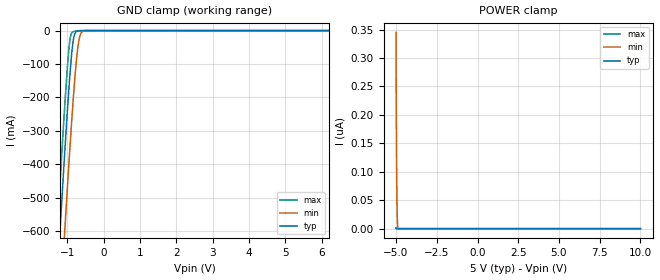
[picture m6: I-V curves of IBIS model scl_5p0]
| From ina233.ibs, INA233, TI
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|   scl_5p0
[Model]   scl_5p0
Model_type   Input
Vinl = 0.4
Vinh = 3.5
|   typ   min   max
C_comp   6.141E-13   5.923E-13   6.345E-13
| Where Nom  PVT is Nominal Process, 5V, 25C
|   Fast PVT is Strong Process,  5.5V, -40C
|   Slow PVT is Weak Process,   4.5V, 125C
[Voltage Range]   5   4.5   5.5
[Temperature Range]   25   125   -40
[Power Clamp Reference]   5   4.5   5.5
[GND Clamp Reference]   0   0   0
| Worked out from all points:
|   GND clamp passes 1 mA (typ) near -0.71 V on its own axis
[GND Clamp]
|   Voltage   I(typ)   I(min)   I(max)
-5V       -8.058A    -8.271A    -7.934A
-1.43V    -1.024A    -1.261A    -882.3mA
-1.25V    -684.6mA   -922.1mA   -542.1mA
-1.235V   -656.8mA   -894.2mA   -514.2mA
-1.175V   -546.3mA   -783.3mA   -404mA
-1.085V   -384.5mA   -619.4mA   -244.5mA
-950mV    -160mA     -382.6mA   -45.51mA
-905mV    -96.55mA   -307.7mA   -13.63mA
-830mV    -23.26mA   -190.7mA   -2.862mA
-695mV    -720.9uA   -36.31mA   -637uA
-515mV    -13.73uA   -522.2uA   -21.3uA
10V       0A         0A         0A
[POWER Clamp]
|   Voltage   I(typ)   I(min)   I(max)
-5V       633pA      344.9nA    1.293nA
-4.985V   316.5pA    207.2nA    646.5pA
-4.97V    0A         128.5nA    0A
-4.955V   0A         77.66nA    0A
-4.94V    0A         44.81nA    0A
-4.925V   0A         23.58nA    0A
-4.91V    0A         9.869nA    0A
-4.895V   0A         1.008nA    0A
-4.865V   0A         0A         0A
10V       0A         0A         0A
